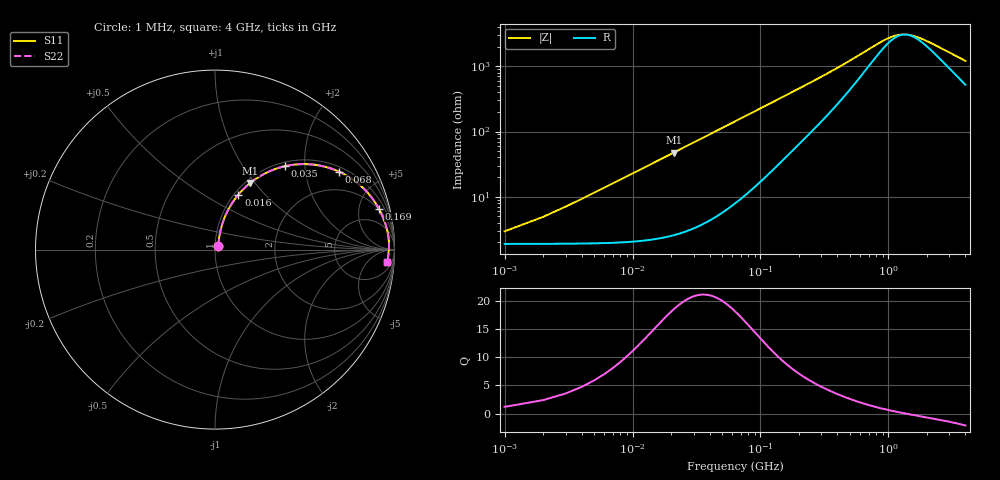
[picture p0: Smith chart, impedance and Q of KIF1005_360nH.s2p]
!version-2
!date-12.2020
!Series
# MHz S RI R 50
!Freq ReS11 ImS11 ReS21 ImS21 ReS12 ImS12 ReS22 ImS22
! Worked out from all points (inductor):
!   4000 points, 1 MHz to 4 GHz, reference 50 ohm
!   read as one part in series: L = 359 nH near 21 MHz
!   highest Q = 18.5 at 21 MHz (marker M1), where L = 359 nH
!   self-resonance near 1.369 GHz
!   S11 on the Smith chart (normalised r, x): 1 MHz: 1.04, +0.05; 16 MHz: 1.05, +0.72; 35 MHz: 1.07, +1.58; 68 MHz: 1.18, +3.07; 169 MHz: 1.92, +7.64; 4 GHz: 11, -22
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1  0.0189 0.0217  0.9811 -0.0217  0.9811 -0.0217  0.0189 0.0217
16  0.1305 0.3069  0.8695 -0.3069  0.8695 -0.3069  0.1305 0.3069
21  0.1964 0.3712  0.8036 -0.3712  0.8036 -0.3712  0.1964 0.3712
27  0.2806 0.4254  0.7194 -0.4254  0.7194 -0.4254  0.2806 0.4254
35  0.3895 0.4645  0.6105 -0.4645  0.6105 -0.4645  0.3895 0.4645
49  0.548 0.4735  0.452 -0.4735  0.452 -0.4735  0.548 0.4735
68  0.6925 0.4337  0.3075 -0.4337  0.3075 -0.4337  0.6925 0.4337
86  0.7761 0.3848  0.2239 -0.3848  0.2239 -0.3848  0.7761 0.3848
107  0.8359 0.3328  0.1641 -0.3328  0.1641 -0.3328  0.8359 0.3328
169  0.9128 0.2285  0.0872 -0.2285  0.0872 -0.2285  0.9128 0.2285
255  0.9458 0.1542  0.0542 -0.1542  0.0542 -0.1542  0.9458 0.1542
366  0.9601 0.1048  0.0399 -0.1048  0.0399 -0.1048  0.9601 0.1048
506  0.9664 0.0704  0.0336 -0.0704  0.0336 -0.0704  0.9664 0.0704
668  0.9689 0.0466  0.0311 -0.0466  0.0311 -0.0466  0.9689 0.0466
837  0.9695 0.0302  0.0305 -0.0302  0.0305 -0.0302  0.9695 0.0302
1000  0.9694 0.0186  0.0306 -0.0186  0.0306 -0.0186  0.9694 0.0186
1161  0.9691 0.00953  0.0309 -0.00953  0.0309 -0.00953  0.9691 0.00953
1334  0.9687 0.00149  0.0313 -0.00149  0.0313 -0.00149  0.9687 0.00149
2001  0.9668 -0.0215  0.0332 0.0215  0.0332 0.0215  0.9668 -0.0215
2667  0.9649 -0.039  0.0351 0.039  0.0351 0.039  0.9649 -0.039
3334  0.963 -0.0545  0.037 0.0545  0.037 0.0545  0.963 -0.0545
4000  0.9609 -0.069  0.0391 0.069  0.0391 0.069  0.9609 -0.069
